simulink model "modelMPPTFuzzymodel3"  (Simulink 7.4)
settings: Solver=ode1  SolverMode=SingleTasking  StartTime=0.0  StopTime=10  FixedStep=1e-4  MaxStep=1e-5
libraries: fuzblock x1

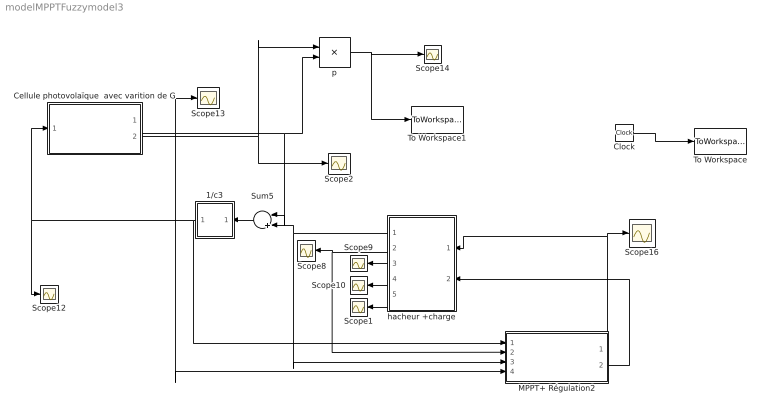
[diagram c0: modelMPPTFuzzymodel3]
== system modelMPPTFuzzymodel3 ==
  1/c3 : Subsystem
  Cellule photovolaïque  avec varition de G : Subsystem  mask{Coc=-152e-3, Csc=1.4e-3, Vmpp=35, Impp=3.15, Voc=43.5, Isc=3.45, Tstc=25, Tc=25, Gstc=1000}
  Clock : Clock
  MPPT+ Régulation2 : Subsystem
  Scope{1..2,8..10,12..14,16} (9 alike) : Scope
  Sum5 : Sum  Inputs=|+-  OutDataType=sfix(16)  OutScaling=2^0
  To Workspace : ToWorkspace  VariableName=t  SampleTime=-1  SaveFormat=Array
  To Workspace1 : ToWorkspace  VariableName=P  SampleTime=-1  SaveFormat=Array
  hacheur +charge : Subsystem
  p : Product  OutDataType=sfix(16)  OutScaling=2^0
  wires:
  1/c3/1(Vdc) -> Scope12/1, Cellule photovolaïque  avec varition de G/1(v), MPPT+ Régulation2/1(vpv)
  Cellule photovolaïque  avec varition de G/1(i+di) -> Scope13/1, MPPT+ Régulation2/4(ipv), p/2, Sum5/1
  hacheur +charge/3(iCH) -> Scope9/1
  hacheur +charge/4(Pch) -> Scope10/1
  hacheur +charge/2(Vch) -> Scope8/1, MPPT+ Régulation2/2(vch)
  MPPT+ Régulation2/1(1-alpha) -> hacheur +charge/1(" 1-alpha"), Scope16/1
  MPPT+ Régulation2/2(VPV1) -> hacheur +charge/2(vpv)
  p/1 -> Scope14/1, To Workspace1/1
  hacheur +charge/5(iL'1) -> Scope1/1
  hacheur +charge/1(iL) -> Sum5/2, MPPT+ Régulation2/3(il)
  Clock/1 -> To Workspace/1
  Sum5/1 -> 1/c3/1(Idc)
  Cellule photovolaïque  avec varition de G/2(V+dV1) -> p/1, Scope2/1

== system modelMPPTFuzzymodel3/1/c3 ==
  Idc : Inport  OutDataType=sfix(16)  OutScaling=2^0
  Gain : Gain  Gain=1/900e-5  ParameterDataType=sfix(16)  ParameterScaling=2^0  OutDataType=sfix(16)  OutScaling=2^0
  Integrator : Integrator
  Vdc : Outport
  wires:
  Gain/1 -> Integrator/1
  Idc/1 -> Gain/1
  Integrator/1 -> Vdc/1

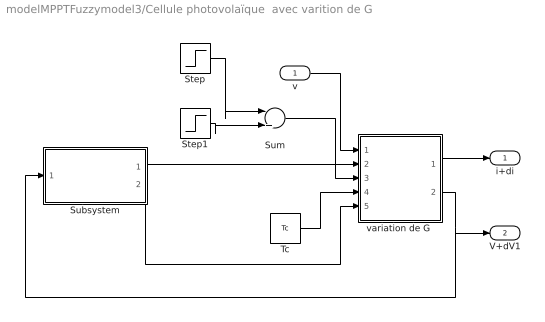
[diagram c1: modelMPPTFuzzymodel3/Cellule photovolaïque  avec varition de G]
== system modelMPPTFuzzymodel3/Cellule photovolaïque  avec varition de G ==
  v : Inport  OutDataType=sfix(16)  OutScaling=2^0
  Step : Step  Time=10  Before=1000  After=900  SampleTime=0
  Step1 : Step  Time=10  After=100  SampleTime=0
  Subsystem : Subsystem
  Sum : Sum  Inputs=|++  OutDataType=sfix(16)  OutScaling=2^0
  Tc : Constant  Value=Tc  OutDataType=sfix(16)  OutScaling=2^0
  "variation de G " : Subsystem
  i+di : Outport
  V+dV1 : Outport  Port=2
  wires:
  Subsystem/1(I1) -> "variation de G "/2(I)
  Tc/1 -> "variation de G "/4(Tc)
  Subsystem/2(np) -> "variation de G "/5(np)
  "variation de G "/1(I+dI2) -> i+di/1
  v/1 -> "variation de G "/1(V)
  "variation de G "/2(V+dV) -> Subsystem/1(V), V+dV1/1
  Step/1 -> Sum/1
  Sum/1 -> "variation de G "/3(G)
  Step1/1 -> Sum/2

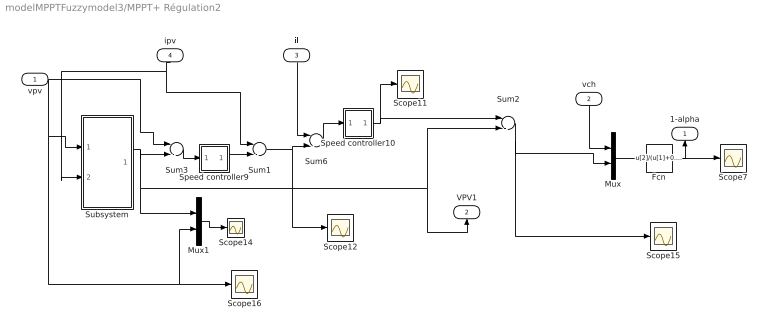
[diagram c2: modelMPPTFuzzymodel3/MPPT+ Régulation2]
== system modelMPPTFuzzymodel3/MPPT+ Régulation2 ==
  vpv : Inport  OutDataType=sfix(16)  OutScaling=2^0
  vch : Inport  Port=2  OutDataType=sfix(16)  OutScaling=2^0
  il : Inport  Port=3  OutDataType=sfix(16)  OutScaling=2^0
  ipv : Inport  Port=4  OutDataType=sfix(16)  OutScaling=2^0
  Fcn : Fcn  Expr=u[2]/(u[1]+0.1)
  Mux : Mux  Inputs=2
  Mux1 : Mux  Inputs=2
  Scope{7,11..12,14..16} (6 alike) : Scope
  Speed controller10 : Subsystem  mask{Kp2=0.01, Ki2=0.1963}
      mask prompts: Kp2 "Proportional gain (Kp)"; Ki2 "Integral gain (Ki)"
      mask help: Proportional-Integral Speed Controller
  Speed controller9 : Subsystem  mask{Kp2=7, Ki2=33.62}
      mask prompts: Kp2 "Proportional gain (Kp)"; Ki2 "Integral gain (Ki)"
      mask help: Proportional-Integral Speed Controller
  Subsystem : Subsystem
  Sum{1..3,6} (4 alike) : Sum  Inputs=|-+  OutDataType=sfix(16)  OutScaling=2^0
  1-alpha : Outport
  VPV1 : Outport  Port=2
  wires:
  Mux1/1 -> Scope14/1
  Subsystem/1(Vref) -> Mux1/1, VPV1/1, Sum2/2, Sum3/2
  Speed controller9/1(Ura) -> Sum1/2
  vpv/1 -> Sum3/1, Scope16/1, Mux1/2, Subsystem/1(Vpv)
  Sum1/1 -> Scope12/1, Sum6/2
  vch/1 -> Mux/1
  Sum2/1 -> Mux/2, Scope15/1
  Fcn/1 -> 1-alpha/1, Scope7/1
  Mux/1 -> Fcn/1
  Speed controller10/1(Ura) -> Sum2/1, Scope11/1
  Sum6/1 -> Speed controller10/1(Ia)
  ipv/1 -> Sum1/1, Subsystem/2(Ipv)
  Sum3/1 -> Speed controller9/1(Ia)
  il/1 -> Sum6/1

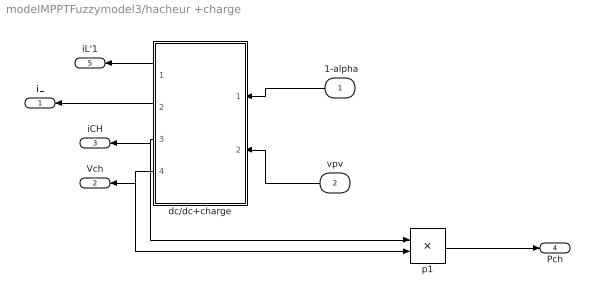
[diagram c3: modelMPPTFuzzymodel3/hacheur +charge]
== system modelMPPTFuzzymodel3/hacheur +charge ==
  " 1-alpha" : Inport  OutDataType=sfix(16)  OutScaling=2^0
  vpv : Inport  Port=2  OutDataType=sfix(16)  OutScaling=2^0
  dc/dc+charge : Subsystem
  p1 : Product  OutDataType=sfix(16)  OutScaling=2^0
  iL : Outport
  Vch : Outport  Port=2
  iCH : Outport  Port=3
  Pch : Outport  Port=4
  iL'1 : Outport  Port=5
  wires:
  vpv/1 -> dc/dc+charge/2(vcpv)
  dc/dc+charge/3(iCH) -> iCH/1, p1/1
  dc/dc+charge/4(Vch) -> Vch/1, p1/2
  p1/1 -> Pch/1
  dc/dc+charge/2(iL) -> iL/1
  " 1-alpha"/1 -> dc/dc+charge/1(1-alpha)
  dc/dc+charge/1(iL'1) -> iL'1/1

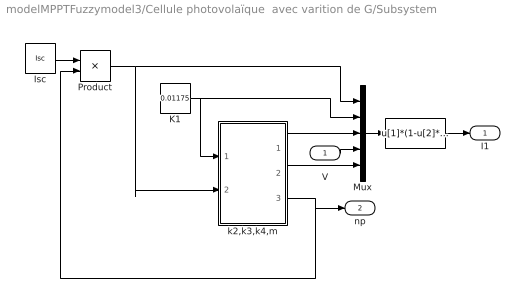
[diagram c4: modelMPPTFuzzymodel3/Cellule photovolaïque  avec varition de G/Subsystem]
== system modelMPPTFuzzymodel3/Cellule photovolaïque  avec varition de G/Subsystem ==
  V : Inport  OutDataType=sfix(16)  OutScaling=2^0
  I : Fcn  Expr=u[1]*(1-u[2]*(exp(u[3]*(u[4]^u[5]))-1))
  Isc : Constant  Value=Isc  OutDataType=sfix(16)  OutScaling=2^0
  K1 : Constant  Value=0.01175  OutDataType=sfix(16)  OutScaling=2^0
  Mux : Mux  Inputs=5
  Product : Product  OutDataType=sfix(16)  OutScaling=2^0
  k2,k3,k4,m : Subsystem
  I1 : Outport
  np : Outport  Port=2
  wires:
  Isc/1 -> Product/1
  K1/1 -> Mux/2, k2,k3,k4,m/1(k1)
  k2,k3,k4,m/1(k2) -> Mux/3
  k2,k3,k4,m/2(m) -> Mux/5
  Mux/1 -> I/1
  V/1 -> Mux/4
  I/1 -> I1/1
  k2,k3,k4,m/3(Np1) -> np/1, Product/2
  Product/1 -> Mux/1, k2,k3,k4,m/2(Isc)

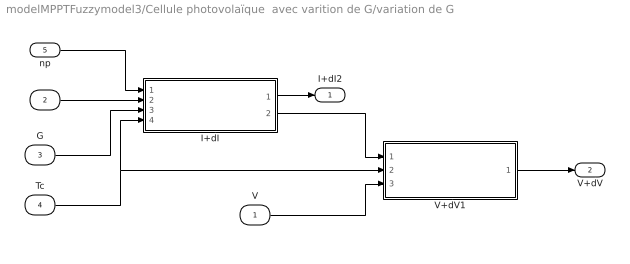
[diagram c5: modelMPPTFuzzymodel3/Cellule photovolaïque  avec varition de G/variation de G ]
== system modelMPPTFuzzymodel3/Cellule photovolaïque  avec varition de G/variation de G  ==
  V : Inport  OutDataType=sfix(16)  OutScaling=2^0
  I : Inport  Port=2  OutDataType=sfix(16)  OutScaling=2^0
  G : Inport  Port=3  OutDataType=sfix(16)  OutScaling=2^0
  Tc : Inport  Port=4  OutDataType=sfix(16)  OutScaling=2^0
  np : Inport  Port=5  OutDataType=sfix(16)  OutScaling=2^0
  I+dI : Subsystem
  V+dV1 : Subsystem
  I+dI2 : Outport
  V+dV : Outport  Port=2
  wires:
  I/1 -> I+dI/2(I)
  I+dI/1(I+dI1) -> I+dI2/1
  V/1 -> V+dV1/3(v)
  I+dI/2(dI) -> V+dV1/1(dI)
  Tc/1 -> I+dI/4(Tc), V+dV1/2(Tc)
  np/1 -> I+dI/1(np)
  G/1 -> I+dI/3(G)
  V+dV1/1(V+dV1) -> V+dV/1

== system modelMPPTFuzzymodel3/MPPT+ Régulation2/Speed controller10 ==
  Ia : Inport  OutDataType=sfix(16)  OutScaling=2^0
  Gain : Gain  Gain=Ki2  ParameterDataType=sfix(16)  ParameterScaling=2^0  OutDataType=sfix(16)  OutScaling=2^0
  Gain3 : Gain  Gain=Kp2  ParameterDataType=sfix(16)  ParameterScaling=2^0  OutDataType=sfix(16)  OutScaling=2^0
  Integrator : Integrator  UpperSaturationLimit=30  LowerSaturationLimit=-30
  Sum2 : Sum  OutDataType=sfix(16)  OutScaling=2^0
  Ura : Outport  InitialOutput=0
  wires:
  Gain/1 -> Integrator/1
  Gain3/1 -> Sum2/1
  Sum2/1 -> Ura/1
  Integrator/1 -> Sum2/2
  Ia/1 -> Gain/1, Gain3/1

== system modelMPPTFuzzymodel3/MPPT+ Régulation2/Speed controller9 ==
  Ia : Inport  OutDataType=sfix(16)  OutScaling=2^0
  Gain : Gain  Gain=Ki2  ParameterDataType=sfix(16)  ParameterScaling=2^0  OutDataType=sfix(16)  OutScaling=2^0
  Gain3 : Gain  Gain=Kp2  ParameterDataType=sfix(16)  ParameterScaling=2^0  OutDataType=sfix(16)  OutScaling=2^0
  Integrator : Integrator  UpperSaturationLimit=30  LowerSaturationLimit=-30
  Sum2 : Sum  OutDataType=sfix(16)  OutScaling=2^0
  Ura : Outport  InitialOutput=0
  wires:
  Ia/1 -> Gain3/1, Gain/1
  Integrator/1 -> Sum2/2
  Sum2/1 -> Ura/1
  Gain3/1 -> Sum2/1
  Gain/1 -> Integrator/1

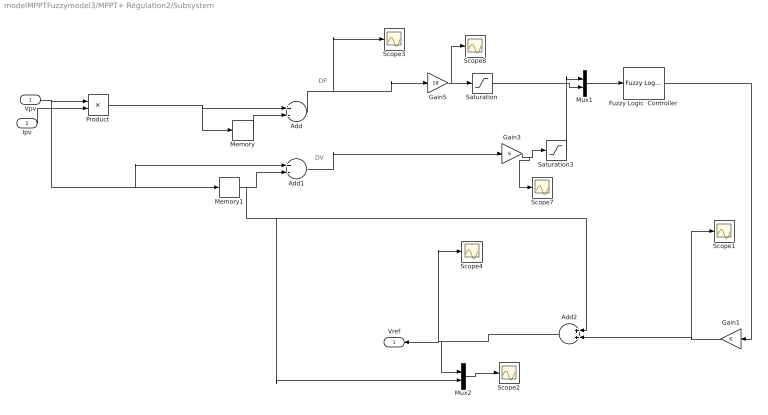
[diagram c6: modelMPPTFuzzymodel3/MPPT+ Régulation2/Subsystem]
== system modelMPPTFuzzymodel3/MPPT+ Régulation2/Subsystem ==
  note: DP
  note: DV
  Vpv : Inport
  Ipv : Inport  Port=2
  Add : Sum  Inputs=+-  OutDataType=sfix(16)  OutScaling=2^-10
  Add1 : Sum  Inputs=+-  OutDataType=sfix(16)  OutScaling=2^-10
  Add2 : Sum  OutDataType=sfix(16)  OutScaling=2^-10
  Fuzzy Logic  Controller : fuzblock/Fuzzy Logic  Controller  SystemSampleTime=-1  fis=SAMM
  Gain1 : Gain  ParameterDataType=sfix(16)  ParameterScaling=2^0  OutDataType=sfix(16)  OutScaling=2^0
  Gain3 : Gain  Gain=6  ParameterDataType=sfix(16)  ParameterScaling=2^0  OutDataType=sfix(16)  OutScaling=2^0
  Gain5 : Gain  Gain=18  ParameterDataType=sfix(16)  ParameterScaling=2^0  OutDataType=sfix(16)  OutScaling=2^0
  Memory : Memory
  Memory1 : Memory
  Mux1 : Mux  Inputs=2
  Mux2 : Mux  Inputs=2
  Product : Product  OutDataType=sfix(16)  OutScaling=2^0
  Saturation : Saturate  UpperLimit=1  LowerLimit=-1  OutDataType=sfix(16)  OutScaling=2^0
  Saturation3 : Saturate  UpperLimit=1  LowerLimit=-1  OutDataType=sfix(16)  OutScaling=2^0
  Scope{1..4,7..8} (6 alike) : Scope
  Vref : Outport  OutDataType=sfix(16)  OutScaling=2^0
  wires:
  Memory/1 -> Add/2
  Memory1/1 -> Add1/2, Add2/1, Mux2/2
  Fuzzy Logic  Controller/1 -> Gain1/1
  Add1/1 -> Gain3/1
  Product/1 -> Add/1, Memory/1
  Add/1 -> Scope3/1, Gain5/1
  Gain5/1 -> Scope8/1, Saturation/1
  Mux1/1 -> Fuzzy Logic  Controller/1
  Gain3/1 -> Scope7/1, Saturation3/1
  Gain1/1 -> Scope1/1, Add2/2
  Vpv/1 -> Memory1/1, Add1/1, Product/1
  Ipv/1 -> Product/2
  Saturation3/1 -> Mux1/1
  Saturation/1 -> Mux1/2
  Add2/1 -> Vref/1, Scope4/1, Mux2/1
  Mux2/1 -> Scope2/1

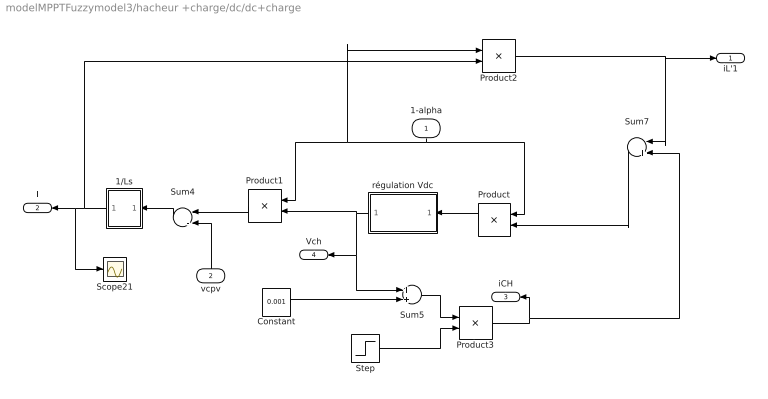
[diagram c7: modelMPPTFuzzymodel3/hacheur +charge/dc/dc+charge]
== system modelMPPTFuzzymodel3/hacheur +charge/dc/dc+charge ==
  1-alpha : Inport  OutDataType=sfix(16)  OutScaling=2^0
  vcpv : Inport  Port=2  OutDataType=sfix(16)  OutScaling=2^0
  1/Ls : Subsystem
  Constant : Constant  Value=0.001  OutDataType=sfix(16)  OutScaling=2^0
  Product : Product  OutDataType=sfix(16)  OutScaling=2^0
  Product1 : Product  OutDataType=sfix(16)  OutScaling=2^0
  Product2 : Product  OutDataType=sfix(16)  OutScaling=2^0
  Product3 : Product  Inputs=/*  OutDataType=sfix(16)  OutScaling=2^0
  Scope21 : Scope
  Step : Step  Before=70  After=70  SampleTime=0
  Sum4 : Sum  Inputs=|-+  OutDataType=sfix(16)  OutScaling=2^0
  Sum5 : Sum  OutDataType=sfix(16)  OutScaling=2^0
  Sum7 : Sum  Inputs=|+-  OutDataType=sfix(16)  OutScaling=2^0
  régulation Vdc : Subsystem
  iL'1 : Outport
  iL : Outport  Port=2
  iCH : Outport  Port=3
  Vch : Outport  Port=4
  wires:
  régulation Vdc/1(Vdc) -> Product1/2, Vch/1, Sum5/1
  Sum7/1 -> Product/2
  1-alpha/1 -> Product/1, Product1/1, Product2/1
  Sum4/1 -> 1/Ls/1(ul)
  vcpv/1 -> Sum4/2
  Product/1 -> régulation Vdc/1(Idc)
  Product1/1 -> Sum4/1
  1/Ls/1(il) -> iL/1, Scope21/1, Product2/2
  Product2/1 -> Sum7/1, iL'1/1
  Step/1 -> Product3/2
  Product3/1 -> iCH/1, Sum7/2
  Sum5/1 -> Product3/1
  Constant/1 -> Sum5/2

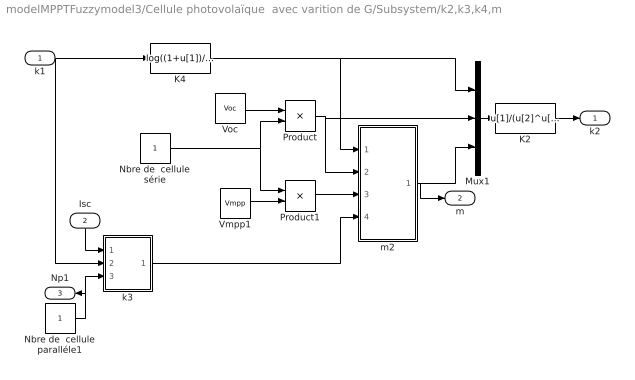
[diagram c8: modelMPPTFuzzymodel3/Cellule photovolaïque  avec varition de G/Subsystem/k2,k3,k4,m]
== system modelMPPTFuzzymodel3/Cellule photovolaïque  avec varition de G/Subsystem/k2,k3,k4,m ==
  k1 : Inport  OutDataType=sfix(16)  OutScaling=2^0
  Isc : Inport  Port=2  OutDataType=sfix(16)  OutScaling=2^0
  K2 : Fcn  Expr=u[1]/(u[2]^u[3])
  K4 : Fcn  Expr=log((1+u[1])/u[1])
  Mux1 : Mux  Inputs=3
  Nbre de  cellule paralléle1 : Constant  OutDataType=sfix(16)  OutScaling=2^0
  Nbre de  cellule série : Constant  OutDataType=sfix(16)  OutScaling=2^0
  Product : Product  OutDataType=sfix(16)  OutScaling=2^0
  Product1 : Product  OutDataType=sfix(16)  OutScaling=2^0
  Vmpp1 : Constant  Value=Vmpp  OutDataType=sfix(16)  OutScaling=2^0
  Voc : Constant  Value=Voc  OutDataType=sfix(16)  OutScaling=2^0
  k3 : Subsystem
  m2 : Subsystem
  k2 : Outport
  m : Outport  Port=2
  Np1 : Outport  Port=3
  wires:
  K4/1 -> Mux1/1, m2/1(k4)
  k1/1 -> K4/1, k3/2(k1)
  m2/1(m) -> Mux1/3, m/1
  Voc/1 -> Product/1
  Nbre de  cellule série/1 -> Product/2, Product1/1
  Product/1 -> Mux1/2, m2/2(Voc)
  Product1/1 -> m2/3(Vmpp)
  Vmpp1/1 -> Product1/2
  Isc/1 -> k3/1(Isc)
  k3/1(k3) -> m2/4("k3 ")
  Nbre de  cellule paralléle1/1 -> k3/3(Np), Np1/1
  Mux1/1 -> K2/1
  K2/1 -> k2/1

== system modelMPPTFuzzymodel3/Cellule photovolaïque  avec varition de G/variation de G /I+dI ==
  np : Inport  OutDataType=sfix(16)  OutScaling=2^0
  I : Inport  Port=2  OutDataType=sfix(16)  OutScaling=2^0
  G : Inport  Port=3  OutDataType=sfix(16)  OutScaling=2^0
  Tc : Inport  Port=4  OutDataType=sfix(16)  OutScaling=2^0
  Gstc : Constant  Value=Gstc  OutDataType=sfix(16)  OutScaling=2^0
  I+dI : Subsystem
  ea4 : Scope
  I+dI1 : Outport
  dI : Outport  Port=2
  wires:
  Tc/1 -> I+dI/4(Tc)
  np/1 -> I+dI/5(np)
  Gstc/1 -> I+dI/3(Gstc)
  G/1 -> I+dI/2(G)
  I/1 -> I+dI/1(I)
  I+dI/2(dI1) -> dI/1
  I+dI/1(I+dI) -> ea4/1, I+dI1/1

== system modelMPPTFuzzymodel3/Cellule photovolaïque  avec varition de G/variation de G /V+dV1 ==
  dI : Inport  OutDataType=sfix(16)  OutScaling=2^0
  Tc : Inport  Port=2  OutDataType=sfix(16)  OutScaling=2^0
  v : Inport  Port=3  OutDataType=sfix(16)  OutScaling=2^0
  V+dV : Subsystem
  ea4 : Scope
  V+dV1 : Outport
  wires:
  dI/1 -> V+dV/2(dI1)
  Tc/1 -> V+dV/3(Tc)
  v/1 -> V+dV/1(V)
  V+dV/1(V+dV) -> ea4/1, V+dV1/1

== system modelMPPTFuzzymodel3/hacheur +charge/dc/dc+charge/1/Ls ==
  ul : Inport  OutDataType=sfix(16)  OutScaling=2^0
  Gain : Gain  Gain=1/0.66e-5  ParameterDataType=sfix(16)  ParameterScaling=2^0  OutDataType=sfix(16)  OutScaling=2^0
  Integrator : Integrator
  il : Outport
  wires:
  Integrator/1 -> il/1
  ul/1 -> Gain/1
  Gain/1 -> Integrator/1

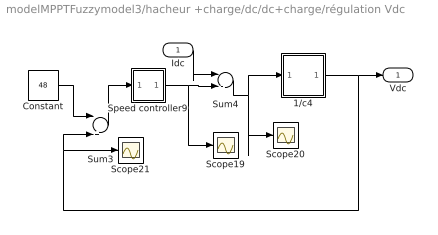
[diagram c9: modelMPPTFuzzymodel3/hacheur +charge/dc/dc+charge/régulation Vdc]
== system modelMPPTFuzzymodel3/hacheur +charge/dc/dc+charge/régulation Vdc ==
  Idc : Inport  OutDataType=sfix(16)  OutScaling=2^0
  1/c4 : Subsystem
  Constant : Constant  Value=48  OutDataType=sfix(16)  OutScaling=2^0
  Scope19 : Scope
  Scope20 : Scope
  Scope21 : Scope
  Speed controller9 : Subsystem  mask{Kp2=98, Ki2=220}
      mask prompts: Kp2 "Proportional gain (Kp)"; Ki2 "Integral gain (Ki)"
      mask help: Proportional-Integral Speed Controller
  Sum3 : Sum  Inputs=|+-  OutDataType=sfix(16)  OutScaling=2^0
  Sum4 : Sum  Inputs=|-+  OutDataType=sfix(16)  OutScaling=2^0
  Vdc : Outport
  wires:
  Sum3/1 -> Speed controller9/1(Ia)
  Constant/1 -> Sum3/1
  Idc/1 -> Sum4/1
  1/c4/1(Vdc) -> Vdc/1, Sum3/2, Scope21/1
  Speed controller9/1(Ura) -> Sum4/2, Scope19/1
  Sum4/1 -> 1/c4/1(Idc), Scope20/1

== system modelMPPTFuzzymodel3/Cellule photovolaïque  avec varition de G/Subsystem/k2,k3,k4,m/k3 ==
  Isc : Inport  OutDataType=sfix(16)  OutScaling=2^0
  k1 : Inport  Port=2  OutDataType=sfix(16)  OutScaling=2^0
  Np : Inport  Port=3  OutDataType=sfix(16)  OutScaling=2^0
  Impp : Constant  Value=Impp  OutDataType=sfix(16)  OutScaling=2^0
  K3 : Fcn  Expr=log((u[1]*(1+u[2])-u[3])/(u[2]*u[1]))
  Mux3 : Mux  Inputs=3
  Product : Product  OutDataType=sfix(16)  OutScaling=2^0
  k3 : Outport
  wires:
  Isc/1 -> Mux3/1
  k1/1 -> Mux3/2
  Np/1 -> Product/2
  Impp/1 -> Product/1
  Mux3/1 -> K3/1
  K3/1 -> k3/1
  Product/1 -> Mux3/3

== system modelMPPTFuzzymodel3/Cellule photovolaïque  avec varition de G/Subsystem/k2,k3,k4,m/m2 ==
  k4 : Inport  OutDataType=sfix(16)  OutScaling=2^0
  Voc : Inport  Port=2  OutDataType=sfix(16)  OutScaling=2^0
  Vmpp : Inport  Port=3  OutDataType=sfix(16)  OutScaling=2^0
  "k3 " : Inport  Port=4  OutDataType=sfix(16)  OutScaling=2^0
  Mux2 : Mux
  m2 : Fcn  Expr=(log(u[1]/u[2]))/(log(u[3]/u[4]))
  m : Outport
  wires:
  Mux2/1 -> m2/1
  k4/1 -> Mux2/2
  Voc/1 -> Mux2/4
  "k3 "/1 -> Mux2/1
  m2/1 -> m/1
  Vmpp/1 -> Mux2/3

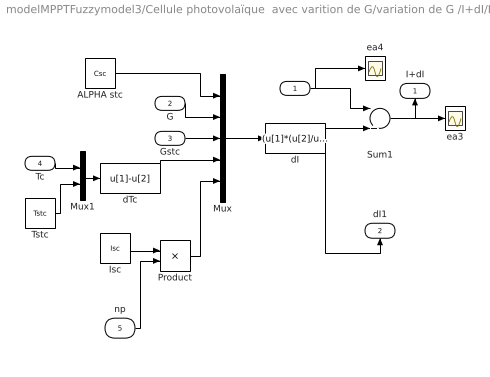
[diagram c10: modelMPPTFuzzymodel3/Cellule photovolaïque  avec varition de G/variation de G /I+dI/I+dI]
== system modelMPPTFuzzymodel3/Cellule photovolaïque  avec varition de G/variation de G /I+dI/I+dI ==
  I : Inport  OutDataType=sfix(16)  OutScaling=2^0
  G : Inport  Port=2  OutDataType=sfix(16)  OutScaling=2^0
  Gstc : Inport  Port=3  OutDataType=sfix(16)  OutScaling=2^0
  Tc : Inport  Port=4  OutDataType=sfix(16)  OutScaling=2^0
  np : Inport  Port=5  OutDataType=sfix(16)  OutScaling=2^0
  ALPHA stc : Constant  Value=Csc  OutDataType=sfix(16)  OutScaling=2^0
  Isc : Constant  Value=Isc  OutDataType=sfix(16)  OutScaling=2^0
  Mux : Mux  Inputs=5
  Mux1 : Mux  Inputs=2
  Product : Product  OutDataType=sfix(16)  OutScaling=2^0
  Sum1 : Sum  Inputs=|++  OutDataType=sfix(16)  OutScaling=2^0
  Tstc : Constant  Value=Tstc  OutDataType=sfix(16)  OutScaling=2^0
  dI : Fcn  Expr=(u[1]*(u[2]/u[3])*u[4])+(((u[2]/u[3])-1)*u[5])
  dTc : Fcn  Expr=u[1]-u[2]
  ea3 : Scope
  ea4 : Scope
  I+dI : Outport
  dI1 : Outport  Port=2
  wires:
  Mux/1 -> dI/1
  ALPHA stc/1 -> Mux/1
  Gstc/1 -> Mux/3
  dTc/1 -> Mux/4
  G/1 -> Mux/2
  Sum1/1 -> ea3/1, I+dI/1
  Mux1/1 -> dTc/1
  Tstc/1 -> Mux1/2
  Tc/1 -> Mux1/1
  I/1 -> Sum1/1, ea4/1
  np/1 -> Product/2
  Isc/1 -> Product/1
  Product/1 -> Mux/5
  dI/1 -> Sum1/2, dI1/1

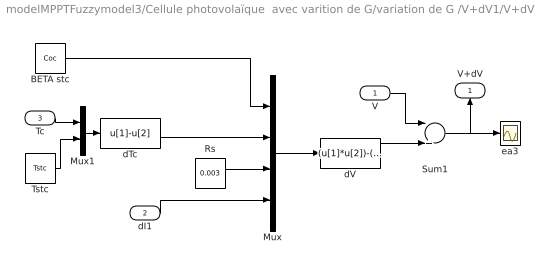
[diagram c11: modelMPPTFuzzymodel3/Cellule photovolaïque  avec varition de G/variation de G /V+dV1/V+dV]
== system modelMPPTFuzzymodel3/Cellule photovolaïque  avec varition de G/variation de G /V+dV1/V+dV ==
  V : Inport  OutDataType=sfix(16)  OutScaling=2^0
  dI1 : Inport  Port=2  OutDataType=sfix(16)  OutScaling=2^0
  Tc : Inport  Port=3  OutDataType=sfix(16)  OutScaling=2^0
  BETA stc : Constant  Value=Coc  OutDataType=sfix(16)  OutScaling=2^0
  Mux : Mux
  Mux1 : Mux  Inputs=2
  Rs : Constant  Value=0.003  OutDataType=sfix(16)  OutScaling=2^0
  Sum1 : Sum  Inputs=|++  OutDataType=sfix(16)  OutScaling=2^0
  Tstc : Constant  Value=Tstc  OutDataType=sfix(16)  OutScaling=2^0
  dTc : Fcn  Expr=u[1]-u[2]
  dV : Fcn  Expr=(u[1]*u[2])-(u[3]*u[4])
  ea3 : Scope
  V+dV : Outport
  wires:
  BETA stc/1 -> Mux/1
  Mux/1 -> dV/1
  dTc/1 -> Mux/2
  Rs/1 -> Mux/3
  dI1/1 -> Mux/4
  Tc/1 -> Mux1/1
  Tstc/1 -> Mux1/2
  Mux1/1 -> dTc/1
  Sum1/1 -> V+dV/1, ea3/1
  V/1 -> Sum1/1
  dV/1 -> Sum1/2

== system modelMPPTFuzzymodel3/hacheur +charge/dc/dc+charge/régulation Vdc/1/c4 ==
  Idc : Inport  OutDataType=sfix(16)  OutScaling=2^0
  Gain : Gain  Gain=1/900e-5  ParameterDataType=sfix(16)  ParameterScaling=2^0  OutDataType=sfix(16)  OutScaling=2^0
  Integrator : Integrator
  Vdc : Outport
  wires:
  Gain/1 -> Integrator/1
  Idc/1 -> Gain/1
  Integrator/1 -> Vdc/1

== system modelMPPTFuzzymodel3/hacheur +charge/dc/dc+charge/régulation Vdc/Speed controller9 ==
  Ia : Inport  OutDataType=sfix(16)  OutScaling=2^0
  Gain : Gain  Gain=Ki2  ParameterDataType=sfix(16)  ParameterScaling=2^0  OutDataType=sfix(16)  OutScaling=2^0
  Gain3 : Gain  Gain=Kp2  ParameterDataType=sfix(16)  ParameterScaling=2^0  OutDataType=sfix(16)  OutScaling=2^0
  Integrator : Integrator  UpperSaturationLimit=30  LowerSaturationLimit=-30
  Sum2 : Sum  OutDataType=sfix(16)  OutScaling=2^0
  Ura : Outport  InitialOutput=0
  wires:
  Ia/1 -> Gain3/1, Gain/1
  Integrator/1 -> Sum2/2
  Sum2/1 -> Ura/1
  Gain3/1 -> Sum2/1
  Gain/1 -> Integrator/1
